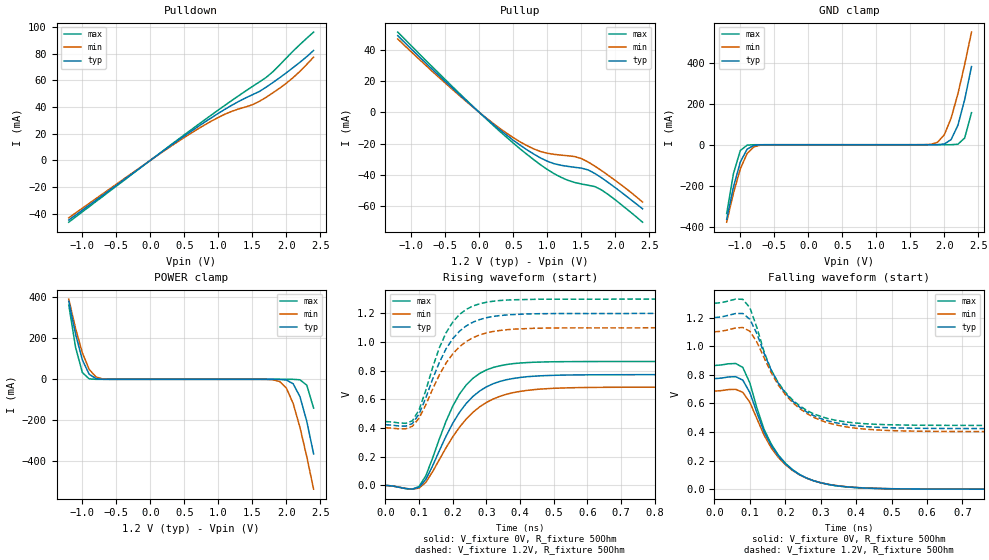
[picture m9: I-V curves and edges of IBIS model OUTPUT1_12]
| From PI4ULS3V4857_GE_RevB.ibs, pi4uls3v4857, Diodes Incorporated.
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[Model]  OUTPUT1_12
Model_type  Output
Vmeas=0.6
|Variable   typ   min   max
C_comp   3.91p   3.89p   3.94p
|Variable   typ   min   max
[Voltage Range]   1.2   1.1   1.3
[Temperature Range]   40   85   -40
[Pullup Reference]   1.2   1.1   1.3
[Pulldown Reference]   0   0   0
[Power Clamp Reference]   1.2   1.1   1.3
[GND Clamp Reference]   0   0   0
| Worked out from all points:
|   slope of the pulldown table from 0 to 0.18 V, typ, clamps not added: 27 ohm
|   slope of the pullup table from 0 to 0.18 V, typ, clamps not added: 26.7 ohm
|   GND clamp passes 1 mA (typ) near -0.72 V on its own axis
|   POWER clamp passes 1 mA (typ) near -0.72 V on its own axis
|   falling waveform, V_fixture 0V, R_fixture 50Ohm: 20-80 % time 103ps typ, 107ps min, 98.2ps max; typ from 0.773 V to 0 V
|   falling waveform, V_fixture 1.2V, R_fixture 50Ohm: 20-80 % time 112ps typ, 121ps min, 104ps max; typ from 1.2 V to 0.423 V
|   rising waveform, V_fixture 0V, R_fixture 50Ohm: 20-80 % time 115ps typ, 130ps min, 99.9ps max; typ from 0 V to 0.773 V
|   rising waveform, V_fixture 1.2V, R_fixture 50Ohm: 20-80 % time 93.9ps typ, 102ps min, 84.2ps max; typ from 0.423 V to 1.2 V
[GND Clamp]
-1.2V     -363mA     -377mA     -335mA
-1.1V     -205mA     -235mA     -140mA
-1V       -84.8mA    -118mA     -28.6mA
-900mV    -21.7mA    -42.8mA    -2.29mA
-800mV    -3.31mA    -10.4mA    -51.5uA
1.7V      183nA      121uA      6.42pA
1.9V      214uA      11.7mA     2.28nA
2V        3.47mA     48.5mA     315nA
2.1V      24.8mA     129mA      39.3uA
2.2V      94.6mA     248mA      2.33mA
2.3V      220mA      391mA      33mA
2.4V      380mA      548mA      156mA
[POWER Clamp]
-1.2V     380mA      391mA      362mA
-1.1V     220mA      248mA      156mA
-1V       94.6mA     129mA      33mA
-900mV    24.8mA     48.5mA     2.33mA
-800mV    3.47mA     11.7mA     39.3uA
-600mV    6.93uA     121uA      2.28nA
1.9V      -256uA     -10.4mA    -3.4nA
2V        -3.31mA    -42.8mA    -455nA
2.1V      -21.7mA    -118mA     -51.5uA
2.2V      -84.8mA    -235mA     -2.29mA
2.3V      -205mA     -377mA     -28.6mA
2.4V      -363mA     -535mA     -140mA
[Pulldown]
| Voltage   I(typ)   I(min)  I(max)
-1.2V     -44.8mA    -43.1mA    -46.4mA
100mV     3.72mA     3.54mA     3.87mA
700mV     25.3mA     23.6mA     26.7mA
1.1V      38.4mA     34.7mA     41.4mA
1.5V      49.2mA     41.7mA     55.4mA
1.7V      54.8mA     47.2mA     62.1mA
1.8V      58.3mA     50.6mA     66.4mA
2.1V      69.6mA     62.1mA     82mA
2.4V      82.4mA     77.4mA     96.2mA
[Pullup]   |Note: Vtable = Vcc - Voutput
| Voltage   I(typ)   I(min)  I(max)
-1.2V     49.2mA     47.1mA     51.5mA
-700mV    28mA       26.6mA     29.6mA
-100mV    3.86mA     3.61mA     4.14mA
300mV     -11.1mA    -10.2mA    -12.1mA
600mV     -21mA      -18.9mA    -23.4mA
800mV     -26.7mA    -23.4mA    -30.3mA
1V        -31.3mA    -26.2mA    -36.6mA
1.3V      -34.6mA    -27.8mA    -43.5mA
1.5V      -35.7mA    -29.6mA    -45.9mA
1.6V      -36.9mA    -31.8mA    -46.7mA
1.8V      -42mA      -37.4mA    -49.8mA
2.4V      -61.8mA    -57.5mA    -70.4mA
[Falling Waveform]
V_fixture = 0V
V_fixture_min = 0V
V_fixture_max = 0V
R_fixture = 50Ohm
C_fixture = 0F
|   Time   V(typ)   V(min)   V(max)
0s        772.6mV    685.5mV    864.5mV
60ps      786.5mV    697.9mV    878.6mV
80ps      762.3mV    676.9mV    851.1mV
100ps     675.4mV    606.8mV    742.1mV
140ps     402.1mV    378.4mV    418.7mV
180ps     233.1mV    222.9mV    239.8mV
240ps     101.9mV    100.5mV    103.3mV
320ps     33.98mV    34.35mV    33.51mV
560ps     1.321mV    1.521mV    1.226mV
1.98ns    0V         0V         0V
[Falling Waveform]
V_fixture = 1.2V
V_fixture_min = 1.1V
V_fixture_max = 1.3V
R_fixture = 50Ohm
C_fixture = 0F
|   Time   V(typ)   V(min)   V(max)
0s        1.2V       1.1V       1.3V
80ps      1.228V     1.13V      1.327V
100ps     1.188V     1.104V     1.269V
120ps     1.085V     1.027V     1.128V
160ps     832.9mV    815.5mV    833.8mV
200ps     671.8mV    661.2mV    677.8mV
260ps     540.7mV    530.4mV    551.5mV
340ps     465.5mV    450.6mV    482.5mV
600ps     425mV      404.5mV    446.7mV
1.98ns    423.4mV    402.3mV    445.4mV
[Rising Waveform]
V_fixture = 0V
V_fixture_min = 0V
V_fixture_max = 0V
R_fixture = 50Ohm
C_fixture = 0F
|   Time   V(typ)   V(min)   V(max)
0s        0V         0V         0V
80ps      -25.91mV   -26.24mV   -25.75mV
100ps     -12.61mV   -18.64mV   -7.326mV
120ps     42.67mV    22.18mV    68.11mV
180ps     343.8mV    263.2mV    448.1mV
220ps     510.4mV    406.6mV    637.9mV
280ps     658.9mV    548.6mV    781.5mV
360ps     737.7mV    636.3mV    843.4mV
580ps     771.1mV    682.6mV    863.9mV
1.98ns    772.6mV    685.5mV    864.5mV
[Rising Waveform]
V_fixture = 1.2V
V_fixture_min = 1.1V
V_fixture_max = 1.3V
R_fixture = 50Ohm
C_fixture = 0F
|   Time   V(typ)   V(min)   V(max)
0s        423.4mV    402.3mV    445.4mV
80ps      431.7mV    412.7mV    450.5mV
100ps     498.8mV    470.2mV    527.7mV
160ps     858.6mV    770.8mV    960.5mV
180ps     952.9mV    853.6mV    1.065V
220ps     1.076V     967.5mV    1.193V
260ps     1.139V     1.031V     1.252V
300ps     1.17V      1.064V     1.278V
520ps     1.199V     1.099V     1.299V
1.98ns    1.2V       1.1V       1.3V
[Ramp]
|   typ   min   max
dV/dt_r   0.63/1.01E-10   0.56/1.05E-10   0.70/0.98E-10
dV/dt_f   0.64/0.80E-10   0.57/0.90E-10   0.71/0.70E-10
R_load =   50.0000
